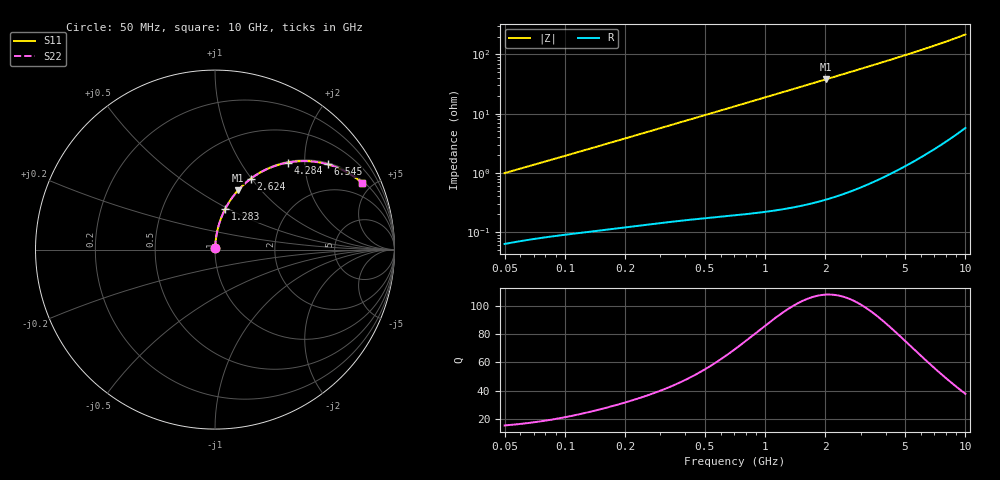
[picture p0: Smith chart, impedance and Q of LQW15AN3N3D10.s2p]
!Murata Part Number: LQW15AN3N3D10
!These Parameters are Measured in Series Mode Connection
!  o--[Z]--o
!Port1  Port2
!  o-------o
!Freq. Start=50[MHz] Stop=10[GHz], 401[Steps]
# Hz S RI R 50
!Freq.(Hz)	S 11(Real)	S 11(Imag)	S 21(Real)	S 21(Imag)	S 12(Real)	S 12(Imag)	S 22(Real)	S 22(Imag)
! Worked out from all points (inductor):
!   401 points, 50 MHz to 10 GHz, reference 50 ohm
!   read as one part in series: L = 3.11 nH near 51.34 MHz
!   highest Q = 108 at 2.013 GHz (marker M1), where L = 3 nH
!   S11 on the Smith chart (normalised r, x): 50 MHz: 1.00, +0.02; 1.283 GHz: 1.00, +0.48; 2.624 GHz: 1.01, +0.99; 4.284 GHz: 1.02, +1.65; 6.545 GHz: 1.04, +2.61; 10 GHz: 1.11, +4.35
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5e7  0.000726 0.00986  0.9993 -0.00986  0.9993 -0.00986  0.000726 0.00986
5.134228e7  0.000742 0.0101  0.9993 -0.0101  0.9993 -0.0101  0.000742 0.0101
1.214486e8  0.00152 0.0233  0.9985 -0.0233  0.9985 -0.0233  0.00152 0.0233
1.956524e8  0.00257 0.0371  0.9974 -0.0371  0.9974 -0.0371  0.00257 0.0371
2.949953e8  0.0045 0.0556  0.9955 -0.0556  0.9955 -0.0556  0.0045 0.0556
4.689809e8  0.00939 0.0875  0.9906 -0.0875  0.9906 -0.0875  0.00939 0.0875
7.071068e8  0.0192 0.1302  0.9808 -0.1302  0.9808 -0.1302  0.0192 0.1302
9.589462e8  0.0334 0.1739  0.9666 -0.1739  0.9666 -0.1739  0.0334 0.1739
1.283367e9  0.0572 0.227  0.9428 -0.227  0.9428 -0.227  0.0572 0.227
1.717543e9  0.097 0.2913  0.903 -0.2913  0.903 -0.2913  0.097 0.2913
2.013439e9  0.1283 0.3299  0.8717 -0.3299  0.8717 -0.3299  0.1283 0.3299
2.298604e9  0.161 0.3629  0.839 -0.3629  0.839 -0.3629  0.161 0.3629
2.624158e9  0.2003 0.3955  0.7997 -0.3955  0.7997 -0.3955  0.2003 0.3955
3.286879e9  0.2833 0.4455  0.7167 -0.4455  0.7167 -0.4455  0.2833 0.4455
4.171863e9  0.3923 0.4825  0.6077 -0.4825  0.6077 -0.4825  0.3923 0.4825
4.283859e9  0.4055 0.4851  0.5945 -0.4851  0.5945 -0.4851  0.4055 0.4851
5.295127e9  0.5159 0.4928  0.4841 -0.4928  0.4841 -0.4928  0.5159 0.4928
6.54512e9  0.6276 0.4751  0.3724 -0.4751  0.3724 -0.4751  0.6276 0.4751
7.37379e9  0.6874 0.4543  0.3126 -0.4543  0.3126 -0.4543  0.6874 0.4543
8.307378e9  0.7431 0.4264  0.2569 -0.4264  0.2569 -0.4264  0.7431 0.4264
9.48396e9  0.7987 0.3888  0.2013 -0.3888  0.2013 -0.3888  0.7987 0.3888
1e10  0.8189 0.3721  0.1811 -0.3721  0.1811 -0.3721  0.8189 0.3721
